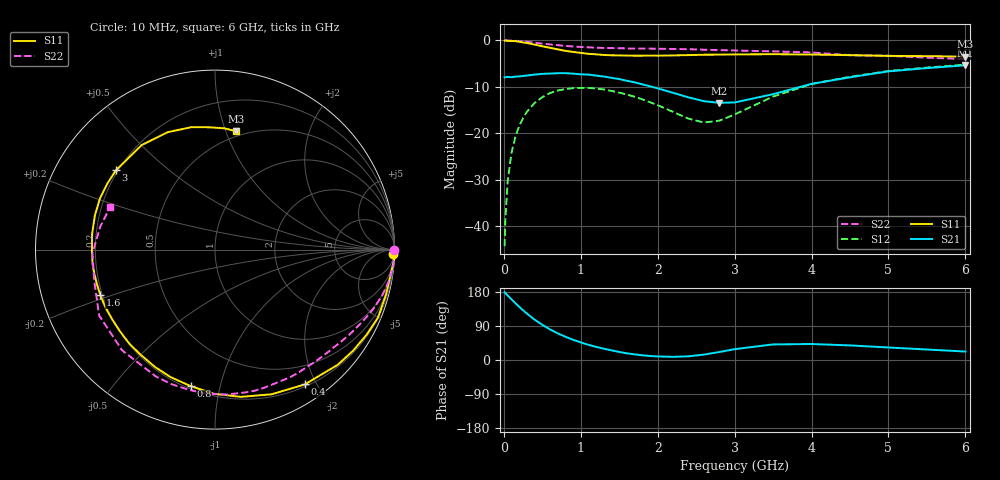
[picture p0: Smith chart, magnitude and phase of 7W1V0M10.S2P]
! Infineon Technologies  Discrete & RF Semiconductors
! BFS17W
! Si NPN RF Bipolar Junction Transistor in SOT323
! VCE = 1 V  IC = 0.1 mA
! Common Emitter S-Parameters:  August  1999
# GHz  S  MA  R  50
!  f  S11  S21  S12  S22
! GHz  MAG  ANG  MAG  ANG  MAG  ANG  MAG  ANG
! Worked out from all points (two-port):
!   36 points, 10 MHz to 6 GHz, reference 50 ohm
!   highest |S21| = -5.35 dB at 6 GHz (marker M1); lowest = -13.4 dB at 2.8 GHz (marker M2)
!   |S21| within 3 dB of the highest: start of sweep to 1.51 GHz; 4.353 GHz to end of sweep
!   lowest |S11| = -3.5 dB at 6 GHz (marker M3), VSWR 5.05, Z = 22.7 + j54.2 ohm
!   |S11| at or under -10 dB: nowhere
!   |S22| runs from -4.0 to 0.0 dB; largest |S21 - S12| = 0.4
!   S11 on the Smith chart (normalised r, x): 10 MHz: 18, -77; 400 MHz: 0.23, -1.85; 800 MHz: 0.22, -0.81; 1.6 GHz: 0.19, -0.18; 3 GHz: 0.19, +0.34; 6 GHz: 0.45, +1.08
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0.01  0.9942 -1.4  0.402 178.8  0.0061 86.1  0.9999 -0.1
0.02  0.9999 -3.1  0.402 176.1  0.0119 87.1  0.9998 -1.1
0.05  0.9891 -7.5  0.405 170.1  0.0308 85.8  0.9982 -2.7
0.1  0.985 -14.5  0.402 160.1  0.0621 80.5  0.9973 -5.3
0.15  0.9842 -22.6  0.408 149.9  0.0917 74.8  0.9896 -7.9
0.2  0.9687 -29.3  0.41 140.3  0.12 70.2  0.9832 -10.4
0.3  0.9378 -43.2  0.419 122.6  0.1707 60.8  0.9662 -15.2
0.4  0.9026 -56.3  0.429 106.5  0.2127 52.0  0.9457 -19.8
0.6  0.833 -80.1  0.44 80.7  0.2716 37.2  0.9061 -27.7
0.8  0.7727 -100.1  0.445 61.4  0.2997 25.2  0.8737 -35.1
1.1  0.7173 -125.4  0.429 40.1  0.3079 11.3  0.8426 -45.4
1.3  0.6978 -139.6  0.409 29.8  0.2969 4.0  0.8297 -52.5
1.6  0.6872 -158.3  0.368 17.6  0.262 -4.1  0.8197 -63.0
2.2  0.6902 172.7  0.273 8.3  0.1701 -4.3  0.8101 -85.4
2.6  0.7017 155.9  0.222 14.2  0.1308 17.4  0.795 -100.6
2.8  0.7036 148.3  0.213 21.0  0.1368 32.4  0.7877 -108.0
3  0.7071 141.2  0.215 28.6  0.1596 43.9  0.78 -114.9
3.5  0.7114 125.0  0.264 41.1  0.2489 53.1  0.7634 -132.7
4  0.7053 111.9  0.341 42.2  0.3396 49.2  0.7425 -150.4
4.5  0.6947 100.9  0.401 38.5  0.4068 42.5  0.6941 -165.9
5.5  0.6777 85.5  0.504 27.7  0.5107 29.6  0.6527 168.9
6  0.6695 80.0  0.54 22.3  0.5495 23.7  0.6301 157.9
